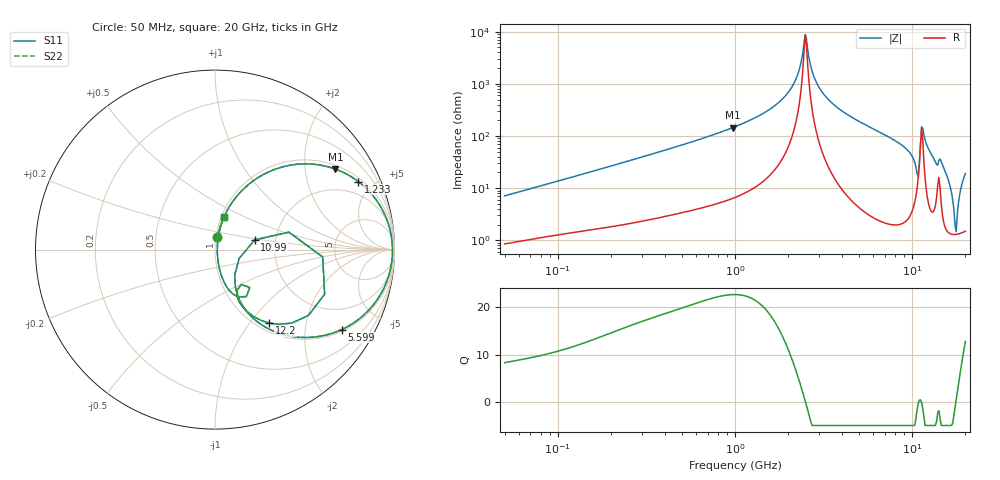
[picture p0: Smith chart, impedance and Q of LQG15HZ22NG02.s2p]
!Murata Part Number: LQG15HZ22NG02
!These Parameters are Measured in Series Mode Connection
!  o--[Z]--o
!Port1  Port2
!  o-------o
!Freq. Start=50[MHz] Stop=20[GHz], 401[Steps]
# Hz S RI R 50
!Freq.(Hz) S11(Real) S11(Imag) S21(Real) S21(Imag) S12(Real) S12(Imag) S22(Real) S22(Imag)
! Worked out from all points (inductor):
!   401 points, 50 MHz to 20 GHz, reference 50 ohm
!   read as one part in series: L = 22.2 nH near 51.52 MHz
!   highest Q = 22.7 at 970.5 MHz (marker M1), where L = 23.7 nH
!   self-resonance near 2.494 GHz
!   S11 on the Smith chart (normalised r, x): 50 MHz: 1.02, +0.14; 1.233 GHz: 1.19, +4.11; 5.599 GHz: 1.06, -3.13; 10.99 GHz: 1.56, +0.18; 12.2 GHz: 1.13, -1.25; 20 GHz: 1.03, +0.38
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5e7  0.0133 0.0692  0.9867 -0.0692  0.9867 -0.0692  0.0133 0.0692
1.364002e8  0.0458 0.1724  0.9542 -0.1724  0.9542 -0.1724  0.0458 0.1724
3.721004e8  0.2093 0.3803  0.7907 -0.3803  0.7907 -0.3803  0.2093 0.3803
9.70487e8  0.6703 0.4486  0.3297 -0.4486  0.3297 -0.4486  0.6703 0.4486
1e9  0.6871 0.4422  0.3129 -0.4422  0.3129 -0.4422  0.6871 0.4422
1.23331e9  0.798 0.3794  0.202 -0.3794  0.202 -0.3794  0.798 0.3794
2.021818e9  0.9694 0.1313  0.0306 -0.1313  0.0306 -0.1313  0.9694 0.1313
2.245319e9  0.9836 0.0673  0.0164 -0.0673  0.0164 -0.0673  0.9836 0.0673
2.493527e9  0.9889 0.00153  0.0111 -0.00153  0.0111 -0.00153  0.9889 0.00153
2.728004e9  0.9863 -0.0555  0.0137 0.0555  0.0137 0.0555  0.9863 -0.0555
3.466789e9  0.9451 -0.2059  0.0549 0.2059  0.0549 0.2059  0.9451 -0.2059
5.598765e9  0.706 -0.4455  0.294 0.4455  0.294 0.4455  0.706 -0.4455
7.442007e9  0.472 -0.4886  0.528 0.4886  0.528 0.4886  0.472 -0.4886
9.745021e9  0.1962 -0.3668  0.8038 0.3668  0.8038 0.3668  0.1962 -0.3668
1.066139e10  0.1104 -0.1396  0.8896 0.1396  0.8896 0.1396  0.1104 -0.1396
1.098561e10  0.2213 0.0542  0.7787 -0.0542  0.7787 -0.0542  0.2213 0.0542
1.149051e10  0.6108 -0.2486  0.3892 0.2486  0.3892 0.2486  0.6108 -0.2486
1.220001e10  0.3023 -0.4094  0.6977 0.4094  0.6977 0.4094  0.3023 -0.4094
1.527346e10  0.0626 -0.2033  0.9374 0.2033  0.9374 0.2033  0.0626 -0.2033
1.646126e10  0.023 -0.0983  0.977 0.0983  0.977 0.0983  0.023 -0.0983
1.747767e10  0.013 -0.0147  0.987 0.0147  0.987 0.0147  0.013 -0.0147
2e10  0.0485 0.1792  0.9515 -0.1792  0.9515 -0.1792  0.0485 0.1792
